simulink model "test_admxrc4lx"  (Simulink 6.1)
settings: Solver=ode45  StartTime=0.0  StopTime=1000  RelTol=1e-3
undefined symbols (not defined in the file or in its folder): Bit, Location, Lower, netlist, Width
libraries: xbsIndex_r3 x86, adlibrary2 x7

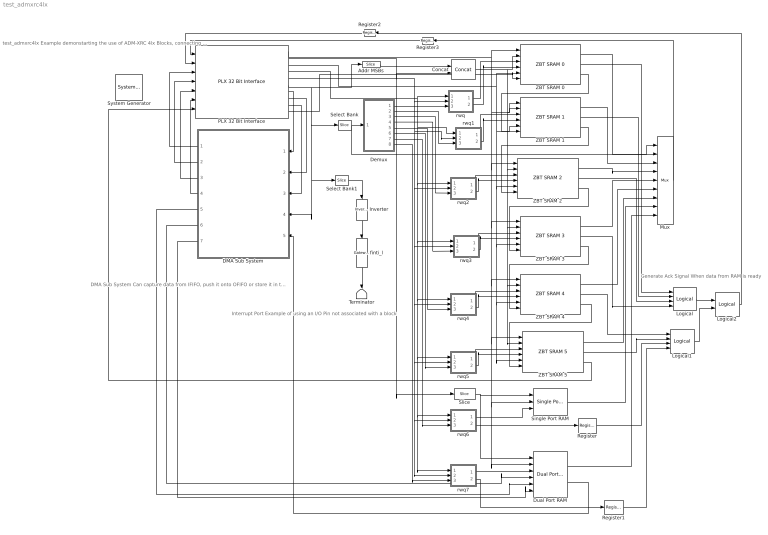
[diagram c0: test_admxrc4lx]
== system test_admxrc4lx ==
  note: test_admxrc4lx Example demonstarting the use of ADM-XRC 4lx Blocks, connecting the Local Bus to ZBT SRAMs and a DMA subsystem
  note: Interrupt Port Example of using an I/O Pin not associated with a block
  note: DMA Sub System Can capture data from IFIFO, push it onto OFIFO or store it in the DP RAM
  note: Generate Ack Signal When data from RAM is ready
  " System Generator" : xbsIndex_r3/ System Generator  Tag=genX  xilinxfamily=Virtex4  part=xc4vlx100  speed=-10  package=ff1148  synthesis_tool=XST  directory=./netlist  testbench=off  simulink_period=1  sysclk_period=10  incr_netlist=off  trim_vbits=Everywhere in SubSystem  dbl_ovrd=According to Block Masks  core_generation=According to Block Masks  run_coregen=off  deprecated_control=off  eval_field=0
  Addr MSBs : xbsIndex_r3/Slice  mode=Lower Bit Location + Width  nbits=5  bit1=0  base1=MSB of Input  bit0=8  base0=LSB of Input  boolean_output=off  explicit_period=off  period=1  dbl_ovrd=off
  Concat : xbsIndex_r3/Concat  num_inputs=2  explicit_period=off  period=1  dbl_ovrd=off
  DMA Sub System : Subsystem  Orientation=left
  Demux : Subsystem
  Dual Port RAM : xbsIndex_r3/Dual Port RAM  depth=1024  initVector=sin(pi*(0:15)/16)  write_mode_A=Read After Write  write_mode_B=Read After Write  latency=1  mem_collision=off  init_zero=on  explicit_period=on  period=1  dbl_ovrd=off  rst_a=off  init_a=0  rst_b=off  init_b=0  show_param=off  distributed_mem=off  use_rpm=off  gen_core=off
  Inverter : xbsIndex_r3/Inverter  Orientation=down  latency=0  explicit_period=off  period=1  en=off  dbl_ovrd=off  show_param=off
  Logical : xbsIndex_r3/Logical  logical_function=OR  inputs=4  precision=Full  arith_type=Unsigned  n_bits=8  bin_pt=2  align_bp=on  latency=0  explicit_period=off  period=1  en=off  dbl_ovrd=off  show_param=off
  Logical1 : xbsIndex_r3/Logical  logical_function=OR  inputs=4  precision=Full  arith_type=Unsigned  n_bits=8  bin_pt=2  align_bp=on  latency=0  explicit_period=off  period=1  en=off  dbl_ovrd=off  show_param=off
  Logical2 : xbsIndex_r3/Logical  logical_function=OR  inputs=2  precision=Full  arith_type=Unsigned  n_bits=8  bin_pt=2  align_bp=on  latency=0  explicit_period=off  period=1  en=off  dbl_ovrd=off  show_param=off
  Mux : xbsIndex_r3/Mux  inputs=8  precision=Full  arith_type="Signed  (2's comp)"  n_bits=8  bin_pt=2  quantization=Truncate  overflow=Wrap  latency=0  explicit_period=off  period=1  en=off  dbl_ovrd=off  show_param=off  mux_type=off  use_rpm=off  gen_core=off
  PLX 32 Bit Interface : adlibrary2/ADM-XRC-II/PLX 32 Bit Interface  program='load test_admxrc2_program.txt'  clock_ratio=1.5
  Register : xbsIndex_r3/Register  init=0  reg_only_valid=off  explicit_period=off  period=1  rst=off  en=off  out_en=off  dbl_ovrd=off  show_param=off
  Register1 : xbsIndex_r3/Register  init=0  reg_only_valid=off  explicit_period=off  period=1  rst=off  en=off  out_en=off  dbl_ovrd=off  show_param=off
  Register2 : xbsIndex_r3/Register  Orientation=left  init=0  reg_only_valid=off  explicit_period=on  period=1  rst=off  en=off  out_en=off  dbl_ovrd=off  show_param=off
  Register3 : xbsIndex_r3/Register  Orientation=left  init=0  reg_only_valid=off  explicit_period=on  period=1  rst=off  en=off  out_en=off  dbl_ovrd=off  show_param=off
  Select Bank : xbsIndex_r3/Slice  mode=Lower Bit Location + Width  nbits=3  bit1=0  base1=MSB of Input  bit0=0  base0=LSB of Input  boolean_output=off  explicit_period=off  period=1  dbl_ovrd=off
  Select Bank1 : xbsIndex_r3/Slice  mode=Lower Bit Location + Width  nbits=1  bit1=0  base1=MSB of Input  bit0=24  base0=LSB of Input  boolean_output=on  explicit_period=off  period=1  dbl_ovrd=off
  Single Port RAM : xbsIndex_r3/Single Port RAM  depth=1024  initVector=sin(pi*(0:15)/16)  write_mode=Read After Write  latency=1  init_zero=on  explicit_period=off  period=1  rst=off  init_reg=0  en=off  dbl_ovrd=off  show_param=off  distributed_mem=off  use_rpm=off  gen_core=off
  Slice : xbsIndex_r3/Slice  mode=Lower Bit Location + Width  nbits=10  bit1=0  base1=MSB of Input  bit0=0  base0=LSB of Input  boolean_output=off  explicit_period=off  period=1  dbl_ovrd=off
  Terminator : Terminator
  ZBT SRAM 0 : adlibrary2/ADM-XRC-4LX//SX/ZBT SRAM 0
  ZBT SRAM 1 : adlibrary2/ADM-XRC-4LX//SX/ZBT SRAM 1
  ZBT SRAM 2 : adlibrary2/ADM-XRC-4LX//SX/ZBT SRAM 2
  ZBT SRAM 3 : adlibrary2/ADM-XRC-4LX//SX/ZBT SRAM 3
  ZBT SRAM 4 : adlibrary2/ADM-XRC-4LX//SX/ZBT SRAM 4
  ZBT SRAM 5 : adlibrary2/ADM-XRC-4LX//SX/ZBT SRAM 5
  finti_l : xbsIndex_r3/Gateway Out  Orientation=down  output_type=Double  nbits=8  bin_pt=6  arith_type=Boolean  quantization=Truncate  overflow=Wrap  hdl_port=on  timing_constraint=None  locs_specified=on  LOCs={'N18'}  needs_fixed_name=off  show_param=off
  rwq : Subsystem
  rwq1 : Subsystem
  rwq2 : Subsystem
  rwq3 : Subsystem
  rwq4 : Subsystem
  rwq5 : Subsystem
  rwq6 : Subsystem
  rwq7 : Subsystem
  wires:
  PLX 32 Bit Interface/1 -> Single Port RAM/2, Dual Port RAM/2, ZBT SRAM 5/1, ZBT SRAM 4/1, ZBT SRAM 3/1, ZBT SRAM 2/1, ZBT SRAM 1/1, ZBT SRAM 0/1
  ZBT SRAM 0/1 -> Mux/2
  ZBT SRAM 1/1 -> Mux/3
  ZBT SRAM 2/1 -> Mux/4
  ZBT SRAM 3/1 -> Mux/5
  ZBT SRAM 4/1 -> Mux/6
  ZBT SRAM 5/1 -> Mux/7
  Single Port RAM/1 -> Mux/8
  Dual Port RAM/1 -> Mux/9
  ZBT SRAM 0/2 -> Logical/1
  ZBT SRAM 1/2 -> Logical/2
  ZBT SRAM 2/2 -> Logical/3
  ZBT SRAM 3/2 -> Logical/4
  ZBT SRAM 4/2 -> Logical1/1
  ZBT SRAM 5/2 -> Logical1/2
  Register/1 -> Logical1/3
  Register1/1 -> Logical1/4
  Mux/1 -> Register3/1
  Logical2/1 -> Register2/1
  Register2/1 -> PLX 32 Bit Interface/2
  Register3/1 -> PLX 32 Bit Interface/1
  Slice/1 -> Single Port RAM/1, Dual Port RAM/1
  Addr MSBs/1 -> Concat/1
  PLX 32 Bit Interface/2 -> Concat/2, Slice/1
  Concat/1 -> ZBT SRAM 4/2, ZBT SRAM 5/2, ZBT SRAM 3/2, ZBT SRAM 2/2, ZBT SRAM 1/2, ZBT SRAM 0/2
  Select Bank/1 -> Demux/1(Select), Mux/1
  rwq2/1(wq) -> ZBT SRAM 2/3
  rwq2/2(rq) -> ZBT SRAM 2/4
  rwq/2(rq) -> ZBT SRAM 0/4
  rwq/1(wq) -> ZBT SRAM 0/3
  rwq3/1(wq) -> ZBT SRAM 3/3
  rwq3/2(rq) -> ZBT SRAM 3/4
  rwq4/1(wq) -> ZBT SRAM 4/3
  rwq4/2(rq) -> ZBT SRAM 4/4
  rwq5/1(wq) -> ZBT SRAM 5/3
  rwq5/2(rq) -> ZBT SRAM 5/4
  rwq6/1(wq) -> Single Port RAM/3
  rwq6/2(rq) -> Register/1
  rwq7/1(wq) -> Dual Port RAM/3
  rwq7/2(rq) -> Register1/1
  Demux/1(En0) -> rwq/3(e)
  Demux/2(En1) -> rwq1/3(e)
  Demux/3(En2) -> rwq2/3(e)
  Demux/4(En3) -> rwq3/3(e)
  Demux/5(En4) -> rwq4/3(e)
  Demux/6(En5) -> rwq5/3(e)
  Demux/7(En6) -> rwq6/3(e)
  Demux/8(En7) -> rwq7/3(e)
  DMA Sub System/1(Status) -> PLX 32 Bit Interface/3
  DMA Sub System/2(Read IFIFO) -> PLX 32 Bit Interface/4
  DMA Sub System/3(Write OFIFO) -> PLX 32 Bit Interface/5
  DMA Sub System/4(OFIFO_Data) -> PLX 32 Bit Interface/6
  Dual Port RAM/2 -> DMA Sub System/5(DP_RAM_Data)
  DMA Sub System/7(DP_RAM_WE) -> Dual Port RAM/6
  DMA Sub System/6(DP_RAM_Addr) -> Dual Port RAM/4
  DMA Sub System/5(DP_RAM_WData) -> Dual Port RAM/5
  Logical/1 -> Logical2/1
  Logical1/1 -> Logical2/2
  Select Bank1/1 -> Inverter/1
  Inverter/1 -> finti_l/1
  finti_l/1 -> Terminator/1
  PLX 32 Bit Interface/9 -> DMA Sub System/3(OFIFO_Full)
  PLX 32 Bit Interface/8 -> DMA Sub System/2(IFIFO_Empty)
  PLX 32 Bit Interface/7 -> DMA Sub System/1(IFIFO_Data)
  PLX 32 Bit Interface/6 -> DMA Sub System/4(Control), Select Bank1/1, Select Bank/1, Addr MSBs/1
  PLX 32 Bit Interface/5 -> rwq/2(r), rwq2/2(r), rwq4/2(r), rwq5/2(r), rwq7/2(r), rwq6/2(r), rwq3/2(r), rwq1/2(r)
  PLX 32 Bit Interface/4 -> rwq/1(w), rwq2/1(w), rwq3/1(w), rwq4/1(w), rwq5/1(w), rwq6/1(w), rwq7/1(w), rwq1/1(w)
  rwq1/1(wq) -> ZBT SRAM 1/3
  rwq1/2(rq) -> ZBT SRAM 1/4
  PLX 32 Bit Interface/3 -> ZBT SRAM 4/5, ZBT SRAM 5/5, ZBT SRAM 3/5, ZBT SRAM 2/5, ZBT SRAM 1/5, ZBT SRAM 0/5
  PLX 32 Bit Interface/10 -> ZBT SRAM 0/6
  ZBT SRAM 0/3 -> ZBT SRAM 1/6
  ZBT SRAM 1/3 -> ZBT SRAM 2/6
  ZBT SRAM 2/3 -> ZBT SRAM 3/6
  ZBT SRAM 3/3 -> ZBT SRAM 4/6
  ZBT SRAM 4/3 -> ZBT SRAM 5/6
  ZBT SRAM 5/3 -> PLX 32 Bit Interface/7

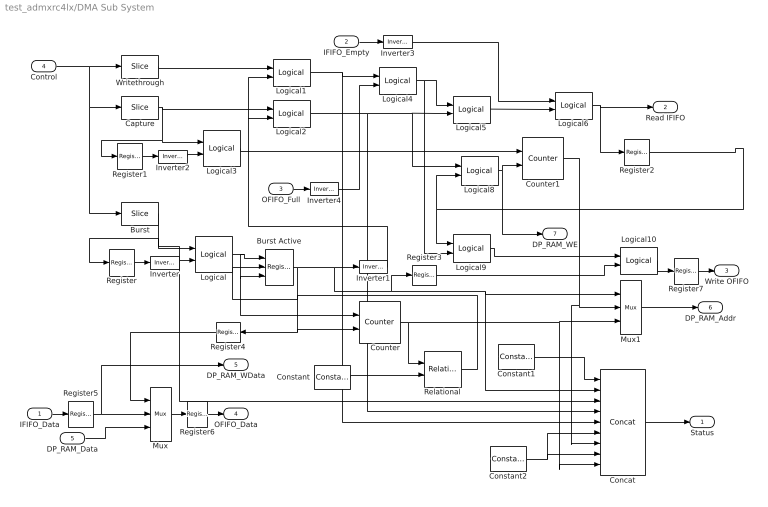
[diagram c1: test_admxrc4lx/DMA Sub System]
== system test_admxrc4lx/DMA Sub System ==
  IFIFO_Data : Inport  Port=1  LatchInput=off
  IFIFO_Empty : Inport  Port=2  LatchInput=off
  OFIFO_Full : Inport  Port=3  LatchInput=off
  Control : Inport  Port=4  LatchInput=off
  DP_RAM_Data : Inport  Port=5  LatchInput=off
  Burst : xbsIndex_r3/Slice  mode=Lower Bit Location + Width  nbits=1  bit1=0  base1=MSB of Input  bit0=18  base0=LSB of Input  boolean_output=on  explicit_period=on  period=1  dbl_ovrd=off
  Burst Active : xbsIndex_r3/Register  init=0  reg_only_valid=off  explicit_period=on  period=1  rst=on  en=on  out_en=off  dbl_ovrd=off  show_param=off
  Capture : xbsIndex_r3/Slice  mode=Lower Bit Location + Width  nbits=1  bit1=0  base1=MSB of Input  bit0=17  base0=LSB of Input  boolean_output=on  explicit_period=on  period=1  dbl_ovrd=off
  Concat : xbsIndex_r3/Concat  num_inputs=9  explicit_period=on  period=1  dbl_ovrd=off
  Constant : xbsIndex_r3/Constant  const=511  equ=P=C  arith_type=Unsigned  n_bits=10  bin_pt=0  opselect=C  inp2=PCIN>>17  opr=+  inp1=P  carry=CIN  iostate=0  explicit_period=off  period=1  dbl_ovrd=off
  Constant1 : xbsIndex_r3/Constant  const=0  equ=P=C  arith_type=Unsigned  n_bits=4  bin_pt=0  opselect=C  inp2=PCIN>>17  opr=+  inp1=P  carry=CIN  iostate=0  explicit_period=off  period=1  dbl_ovrd=off
  Constant2 : xbsIndex_r3/Constant  const=0  equ=P=C  arith_type=Unsigned  n_bits=2  bin_pt=0  opselect=C  inp2=PCIN>>17  opr=+  inp1=P  carry=CIN  iostate=0  explicit_period=off  period=1  dbl_ovrd=off
  Counter : xbsIndex_r3/Counter  cnt_type=Count Limited  n_bits=10  bin_pt=0  arith_type=Unsigned  start_count=0  cnt_to=Inf  cnt_by_val=1  operation=Up  explicit_period=on  period=1  load_pin=off  rst=on  en=on  dbl_ovrd=off  show_param=off  use_rpm=on  gen_core=off
  Counter1 : xbsIndex_r3/Counter  cnt_type=Count Limited  n_bits=10  bin_pt=0  arith_type=Unsigned  start_count=0  cnt_to=Inf  cnt_by_val=1  operation=Up  explicit_period=on  period=1  load_pin=off  rst=on  en=on  dbl_ovrd=off  show_param=off  use_rpm=on  gen_core=off
  Inverter{,1..2,4} (4 alike) : xbsIndex_r3/Inverter  latency=0  explicit_period=off  period=1  en=off  dbl_ovrd=off  show_param=off
  Inverter3 : xbsIndex_r3/Inverter  latency=0  explicit_period=on  period=1  en=off  dbl_ovrd=off  show_param=off
  Logical : xbsIndex_r3/Logical  logical_function=AND  inputs=2  precision=Full  arith_type=Unsigned  n_bits=8  bin_pt=2  align_bp=on  latency=0  explicit_period=on  period=1  en=off  dbl_ovrd=off  show_param=off
  Logical{1..2,4,8..9} (5 alike) : xbsIndex_r3/Logical  logical_function=AND  inputs=2  precision=Full  arith_type=Unsigned  n_bits=8  bin_pt=2  align_bp=on  latency=0  explicit_period=off  period=1  en=off  dbl_ovrd=off  show_param=off
  Logical10 : xbsIndex_r3/Logical  logical_function=OR  inputs=2  precision=Full  arith_type=Unsigned  n_bits=8  bin_pt=2  align_bp=on  latency=0  explicit_period=on  period=1  en=off  dbl_ovrd=off  show_param=off
  Logical3 : xbsIndex_r3/Logical  logical_function=AND  inputs=2  precision=Full  arith_type=Unsigned  n_bits=8  bin_pt=2  align_bp=on  latency=0  explicit_period=on  period=1  en=off  dbl_ovrd=off  show_param=off
  Logical5 : xbsIndex_r3/Logical  logical_function=OR  inputs=2  precision=Full  arith_type=Unsigned  n_bits=8  bin_pt=2  align_bp=on  latency=0  explicit_period=off  period=1  en=off  dbl_ovrd=off  show_param=off
  Logical6 : xbsIndex_r3/Logical  logical_function=AND  inputs=2  precision=Full  arith_type=Unsigned  n_bits=8  bin_pt=2  align_bp=on  latency=0  explicit_period=on  period=1  en=off  dbl_ovrd=off  show_param=off
  Mux : xbsIndex_r3/Mux  inputs=2  precision=Full  arith_type="Signed  (2's comp)"  n_bits=8  bin_pt=2  quantization=Truncate  overflow=Wrap  latency=0  explicit_period=on  period=1  en=off  dbl_ovrd=off  show_param=off  mux_type=off  use_rpm=off  gen_core=off
  Mux1 : xbsIndex_r3/Mux  inputs=2  precision=Full  arith_type="Signed  (2's comp)"  n_bits=8  bin_pt=2  quantization=Truncate  overflow=Wrap  latency=0  explicit_period=off  period=1  en=off  dbl_ovrd=off  show_param=off  mux_type=off  use_rpm=off  gen_core=off
  Register{,1..3,5..7} (7 alike) : xbsIndex_r3/Register  init=0  reg_only_valid=off  explicit_period=on  period=1  rst=off  en=off  out_en=off  dbl_ovrd=off  show_param=off
  Register4 : xbsIndex_r3/Register  Orientation=left  init=0  reg_only_valid=off  explicit_period=on  period=1  rst=off  en=off  out_en=off  dbl_ovrd=off  show_param=off
  Relational : xbsIndex_r3/Relational  mode=a=b  latency=0  explicit_period=off  period=1  en=off  dbl_ovrd=off  show_param=off
  Writethrough : xbsIndex_r3/Slice  mode=Lower Bit Location + Width  nbits=1  bit1=0  base1=MSB of Input  bit0=16  base0=LSB of Input  boolean_output=on  explicit_period=on  period=1  dbl_ovrd=off
  Status : Outport
  Read IFIFO : Outport  Port=2
  Write OFIFO : Outport  Port=3
  OFIFO_Data : Outport  Port=4
  DP_RAM_WData : Outport  Port=5
  DP_RAM_Addr : Outport  Port=6
  DP_RAM_WE : Outport  Port=7
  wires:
  Mux/1 -> Register6/1
  IFIFO_Data/1 -> Register5/1
  DP_RAM_Data/1 -> Mux/3
  Control/1 -> Writethrough/1, Burst/1, Capture/1
  Burst/1 -> Register/1, Logical/1, Concat/3
  Register/1 -> Inverter/1
  Inverter/1 -> Logical/2
  Logical/1 -> Burst Active/1, Burst Active/3, Counter/1
  Burst Active/1 -> Inverter1/1, Register3/1, Mux1/1, Concat/2, Counter/2, Register4/1
  Inverter1/1 -> Logical1/2, Logical2/2
  Capture/1 -> Logical2/1, Logical3/1, Register1/1
  Writethrough/1 -> Logical1/1
  Register1/1 -> Inverter2/1
  Inverter2/1 -> Logical3/2
  Logical3/1 -> Counter1/1
  IFIFO_Empty/1 -> Inverter3/1
  OFIFO_Full/1 -> Inverter4/1
  Logical1/1 -> Logical4/1, Concat/5
  Inverter4/1 -> Logical4/2
  Logical2/1 -> Logical5/2, Logical8/1, Concat/4
  Logical4/1 -> Logical5/1, Logical9/2
  Inverter3/1 -> Logical6/1
  Logical5/1 -> Logical6/2
  Logical6/1 -> Read IFIFO/1, Register2/1
  Register2/1 -> Logical8/2, Logical9/1
  Logical8/1 -> Counter1/2, DP_RAM_WE/1
  Mux1/1 -> DP_RAM_Addr/1
  Counter1/1 -> Mux1/2, Concat/7
  Counter/1 -> Relational/1, Mux1/3, Concat/9
  Logical9/1 -> Logical10/1
  Register3/1 -> Logical10/2
  Constant/1 -> Relational/2
  Relational/1 -> Burst Active/2
  Constant2/1 -> Concat/8, Concat/6
  Concat/1 -> Status/1
  Constant1/1 -> Concat/1
  Logical10/1 -> Register7/1
  Register4/1 -> Mux/1
  Register5/1 -> Mux/2, DP_RAM_WData/1
  Register6/1 -> OFIFO_Data/1
  Register7/1 -> Write OFIFO/1

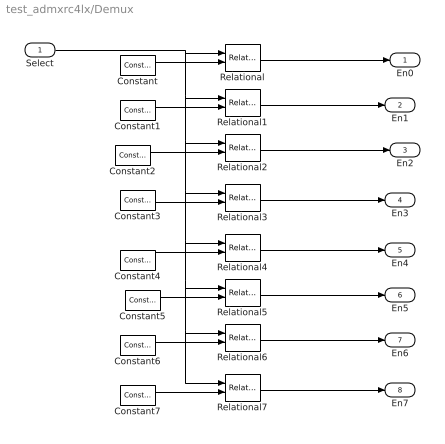
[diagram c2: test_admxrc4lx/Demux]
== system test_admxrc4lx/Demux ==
  Select : Inport  Port=1  LatchInput=off
  Constant : xbsIndex_r3/Constant  const=0  equ=P=C  arith_type=Unsigned  n_bits=3  bin_pt=0  opselect=C  inp2=PCIN>>17  opr=+  inp1=P  carry=CIN  iostate=0  explicit_period=off  period=1  dbl_ovrd=off
  Constant1 : xbsIndex_r3/Constant  const=1  equ=P=C  arith_type=Unsigned  n_bits=3  bin_pt=0  opselect=C  inp2=PCIN>>17  opr=+  inp1=P  carry=CIN  iostate=0  explicit_period=off  period=1  dbl_ovrd=off
  Constant2 : xbsIndex_r3/Constant  const=2  equ=P=C  arith_type=Unsigned  n_bits=3  bin_pt=0  opselect=C  inp2=PCIN>>17  opr=+  inp1=P  carry=CIN  iostate=0  explicit_period=off  period=1  dbl_ovrd=off
  Constant3 : xbsIndex_r3/Constant  const=3  equ=P=C  arith_type=Unsigned  n_bits=3  bin_pt=0  opselect=C  inp2=PCIN>>17  opr=+  inp1=P  carry=CIN  iostate=0  explicit_period=off  period=1  dbl_ovrd=off
  Constant4 : xbsIndex_r3/Constant  const=4  equ=P=C  arith_type=Unsigned  n_bits=3  bin_pt=0  opselect=C  inp2=PCIN>>17  opr=+  inp1=P  carry=CIN  iostate=0  explicit_period=off  period=1  dbl_ovrd=off
  Constant5 : xbsIndex_r3/Constant  const=5  equ=P=C  arith_type=Unsigned  n_bits=3  bin_pt=0  opselect=C  inp2=PCIN>>17  opr=+  inp1=P  carry=CIN  iostate=0  explicit_period=off  period=1  dbl_ovrd=off
  Constant6 : xbsIndex_r3/Constant  const=6  equ=P=C  arith_type=Unsigned  n_bits=3  bin_pt=0  opselect=C  inp2=PCIN>>17  opr=+  inp1=P  carry=CIN  iostate=0  explicit_period=off  period=1  dbl_ovrd=off
  Constant7 : xbsIndex_r3/Constant  const=7  equ=P=C  arith_type=Unsigned  n_bits=3  bin_pt=0  opselect=C  inp2=PCIN>>17  opr=+  inp1=P  carry=CIN  iostate=0  explicit_period=off  period=1  dbl_ovrd=off
  Relational{,1..7} (8 alike) : xbsIndex_r3/Relational  mode=a=b  latency=0  explicit_period=off  period=1  en=off  dbl_ovrd=off  show_param=off
  En0 : Outport
  En1 : Outport  Port=2
  En2 : Outport  Port=3
  En3 : Outport  Port=4
  En4 : Outport  Port=5
  En5 : Outport  Port=6
  En6 : Outport  Port=7
  En7 : Outport  Port=8
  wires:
  Relational/1 -> En0/1
  Relational1/1 -> En1/1
  Relational2/1 -> En2/1
  Relational3/1 -> En3/1
  Relational4/1 -> En4/1
  Relational5/1 -> En5/1
  Relational6/1 -> En6/1
  Relational7/1 -> En7/1
  Select/1 -> Relational/1, Relational1/1, Relational2/1, Relational3/1, Relational4/1, Relational5/1, Relational6/1, Relational7/1
  Constant/1 -> Relational/2
  Constant1/1 -> Relational1/2
  Constant2/1 -> Relational2/2
  Constant3/1 -> Relational3/2
  Constant4/1 -> Relational4/2
  Constant5/1 -> Relational5/2
  Constant6/1 -> Relational6/2
  Constant7/1 -> Relational7/2

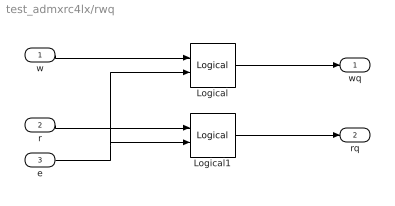
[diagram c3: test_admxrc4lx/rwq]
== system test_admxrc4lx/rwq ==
  w : Inport  Port=1  LatchInput=off
  r : Inport  Port=2  LatchInput=off
  e : Inport  Port=3  LatchInput=off
  Logical : xbsIndex_r3/Logical  logical_function=AND  inputs=2  precision=Full  arith_type=Unsigned  n_bits=8  bin_pt=2  align_bp=on  latency=0  explicit_period=off  period=1  en=off  dbl_ovrd=off  show_param=off
  Logical1 : xbsIndex_r3/Logical  logical_function=AND  inputs=2  precision=Full  arith_type=Unsigned  n_bits=8  bin_pt=2  align_bp=on  latency=0  explicit_period=off  period=1  en=off  dbl_ovrd=off  show_param=off
  wq : Outport
  rq : Outport  Port=2
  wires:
  e/1 -> Logical1/2, Logical/2
  r/1 -> Logical1/1
  w/1 -> Logical/1
  Logical/1 -> wq/1
  Logical1/1 -> rq/1

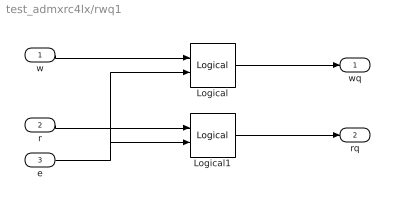
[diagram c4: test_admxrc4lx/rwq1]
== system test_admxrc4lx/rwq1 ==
  w : Inport  Port=1  LatchInput=off
  r : Inport  Port=2  LatchInput=off
  e : Inport  Port=3  LatchInput=off
  Logical : xbsIndex_r3/Logical  logical_function=AND  inputs=2  precision=Full  arith_type=Unsigned  n_bits=8  bin_pt=2  align_bp=on  latency=0  explicit_period=off  period=1  en=off  dbl_ovrd=off  show_param=off
  Logical1 : xbsIndex_r3/Logical  logical_function=AND  inputs=2  precision=Full  arith_type=Unsigned  n_bits=8  bin_pt=2  align_bp=on  latency=0  explicit_period=off  period=1  en=off  dbl_ovrd=off  show_param=off
  wq : Outport
  rq : Outport  Port=2
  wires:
  e/1 -> Logical1/2, Logical/2
  r/1 -> Logical1/1
  w/1 -> Logical/1
  Logical/1 -> wq/1
  Logical1/1 -> rq/1

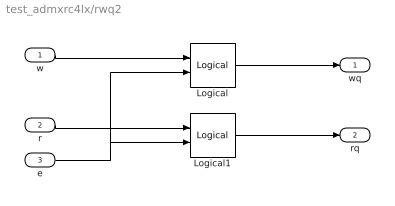
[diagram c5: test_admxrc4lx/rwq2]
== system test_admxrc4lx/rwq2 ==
  w : Inport  Port=1  LatchInput=off
  r : Inport  Port=2  LatchInput=off
  e : Inport  Port=3  LatchInput=off
  Logical : xbsIndex_r3/Logical  logical_function=AND  inputs=2  precision=Full  arith_type=Unsigned  n_bits=8  bin_pt=2  align_bp=on  latency=0  explicit_period=off  period=1  en=off  dbl_ovrd=off  show_param=off
  Logical1 : xbsIndex_r3/Logical  logical_function=AND  inputs=2  precision=Full  arith_type=Unsigned  n_bits=8  bin_pt=2  align_bp=on  latency=0  explicit_period=off  period=1  en=off  dbl_ovrd=off  show_param=off
  wq : Outport
  rq : Outport  Port=2
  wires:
  e/1 -> Logical1/2, Logical/2
  r/1 -> Logical1/1
  w/1 -> Logical/1
  Logical/1 -> wq/1
  Logical1/1 -> rq/1

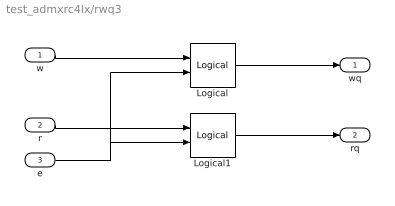
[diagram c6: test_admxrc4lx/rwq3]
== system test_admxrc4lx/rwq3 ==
  w : Inport  Port=1  LatchInput=off
  r : Inport  Port=2  LatchInput=off
  e : Inport  Port=3  LatchInput=off
  Logical : xbsIndex_r3/Logical  logical_function=AND  inputs=2  precision=Full  arith_type=Unsigned  n_bits=8  bin_pt=2  align_bp=on  latency=0  explicit_period=off  period=1  en=off  dbl_ovrd=off  show_param=off
  Logical1 : xbsIndex_r3/Logical  logical_function=AND  inputs=2  precision=Full  arith_type=Unsigned  n_bits=8  bin_pt=2  align_bp=on  latency=0  explicit_period=off  period=1  en=off  dbl_ovrd=off  show_param=off
  wq : Outport
  rq : Outport  Port=2
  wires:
  e/1 -> Logical1/2, Logical/2
  r/1 -> Logical1/1
  w/1 -> Logical/1
  Logical/1 -> wq/1
  Logical1/1 -> rq/1

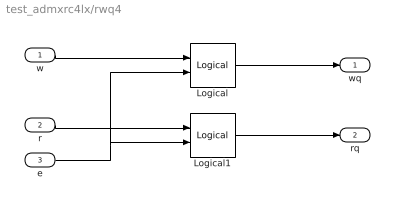
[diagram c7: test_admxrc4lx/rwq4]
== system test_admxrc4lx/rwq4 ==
  w : Inport  Port=1  LatchInput=off
  r : Inport  Port=2  LatchInput=off
  e : Inport  Port=3  LatchInput=off
  Logical : xbsIndex_r3/Logical  logical_function=AND  inputs=2  precision=Full  arith_type=Unsigned  n_bits=8  bin_pt=2  align_bp=on  latency=0  explicit_period=off  period=1  en=off  dbl_ovrd=off  show_param=off
  Logical1 : xbsIndex_r3/Logical  logical_function=AND  inputs=2  precision=Full  arith_type=Unsigned  n_bits=8  bin_pt=2  align_bp=on  latency=0  explicit_period=off  period=1  en=off  dbl_ovrd=off  show_param=off
  wq : Outport
  rq : Outport  Port=2
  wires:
  e/1 -> Logical1/2, Logical/2
  r/1 -> Logical1/1
  w/1 -> Logical/1
  Logical/1 -> wq/1
  Logical1/1 -> rq/1

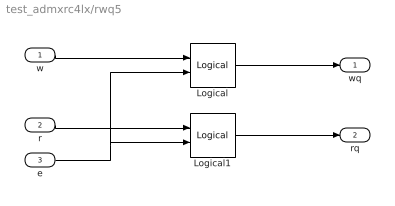
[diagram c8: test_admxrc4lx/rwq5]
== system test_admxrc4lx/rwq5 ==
  w : Inport  Port=1  LatchInput=off
  r : Inport  Port=2  LatchInput=off
  e : Inport  Port=3  LatchInput=off
  Logical : xbsIndex_r3/Logical  logical_function=AND  inputs=2  precision=Full  arith_type=Unsigned  n_bits=8  bin_pt=2  align_bp=on  latency=0  explicit_period=off  period=1  en=off  dbl_ovrd=off  show_param=off
  Logical1 : xbsIndex_r3/Logical  logical_function=AND  inputs=2  precision=Full  arith_type=Unsigned  n_bits=8  bin_pt=2  align_bp=on  latency=0  explicit_period=off  period=1  en=off  dbl_ovrd=off  show_param=off
  wq : Outport
  rq : Outport  Port=2
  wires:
  e/1 -> Logical1/2, Logical/2
  r/1 -> Logical1/1
  w/1 -> Logical/1
  Logical/1 -> wq/1
  Logical1/1 -> rq/1

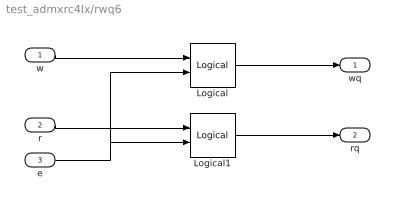
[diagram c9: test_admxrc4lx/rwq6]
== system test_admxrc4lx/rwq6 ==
  w : Inport  Port=1  LatchInput=off
  r : Inport  Port=2  LatchInput=off
  e : Inport  Port=3  LatchInput=off
  Logical : xbsIndex_r3/Logical  logical_function=AND  inputs=2  precision=Full  arith_type=Unsigned  n_bits=8  bin_pt=2  align_bp=on  latency=0  explicit_period=off  period=1  en=off  dbl_ovrd=off  show_param=off
  Logical1 : xbsIndex_r3/Logical  logical_function=AND  inputs=2  precision=Full  arith_type=Unsigned  n_bits=8  bin_pt=2  align_bp=on  latency=0  explicit_period=off  period=1  en=off  dbl_ovrd=off  show_param=off
  wq : Outport
  rq : Outport  Port=2
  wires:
  e/1 -> Logical1/2, Logical/2
  r/1 -> Logical1/1
  w/1 -> Logical/1
  Logical/1 -> wq/1
  Logical1/1 -> rq/1

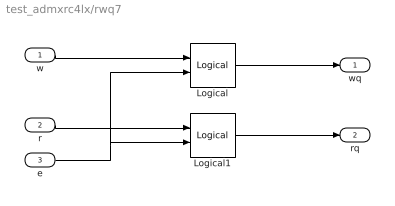
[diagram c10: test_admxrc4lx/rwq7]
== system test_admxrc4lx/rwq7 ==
  w : Inport  Port=1  LatchInput=off
  r : Inport  Port=2  LatchInput=off
  e : Inport  Port=3  LatchInput=off
  Logical : xbsIndex_r3/Logical  logical_function=AND  inputs=2  precision=Full  arith_type=Unsigned  n_bits=8  bin_pt=2  align_bp=on  latency=0  explicit_period=off  period=1  en=off  dbl_ovrd=off  show_param=off
  Logical1 : xbsIndex_r3/Logical  logical_function=AND  inputs=2  precision=Full  arith_type=Unsigned  n_bits=8  bin_pt=2  align_bp=on  latency=0  explicit_period=off  period=1  en=off  dbl_ovrd=off  show_param=off
  wq : Outport
  rq : Outport  Port=2
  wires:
  e/1 -> Logical1/2, Logical/2
  r/1 -> Logical1/1
  w/1 -> Logical/1
  Logical/1 -> wq/1
  Logical1/1 -> rq/1
